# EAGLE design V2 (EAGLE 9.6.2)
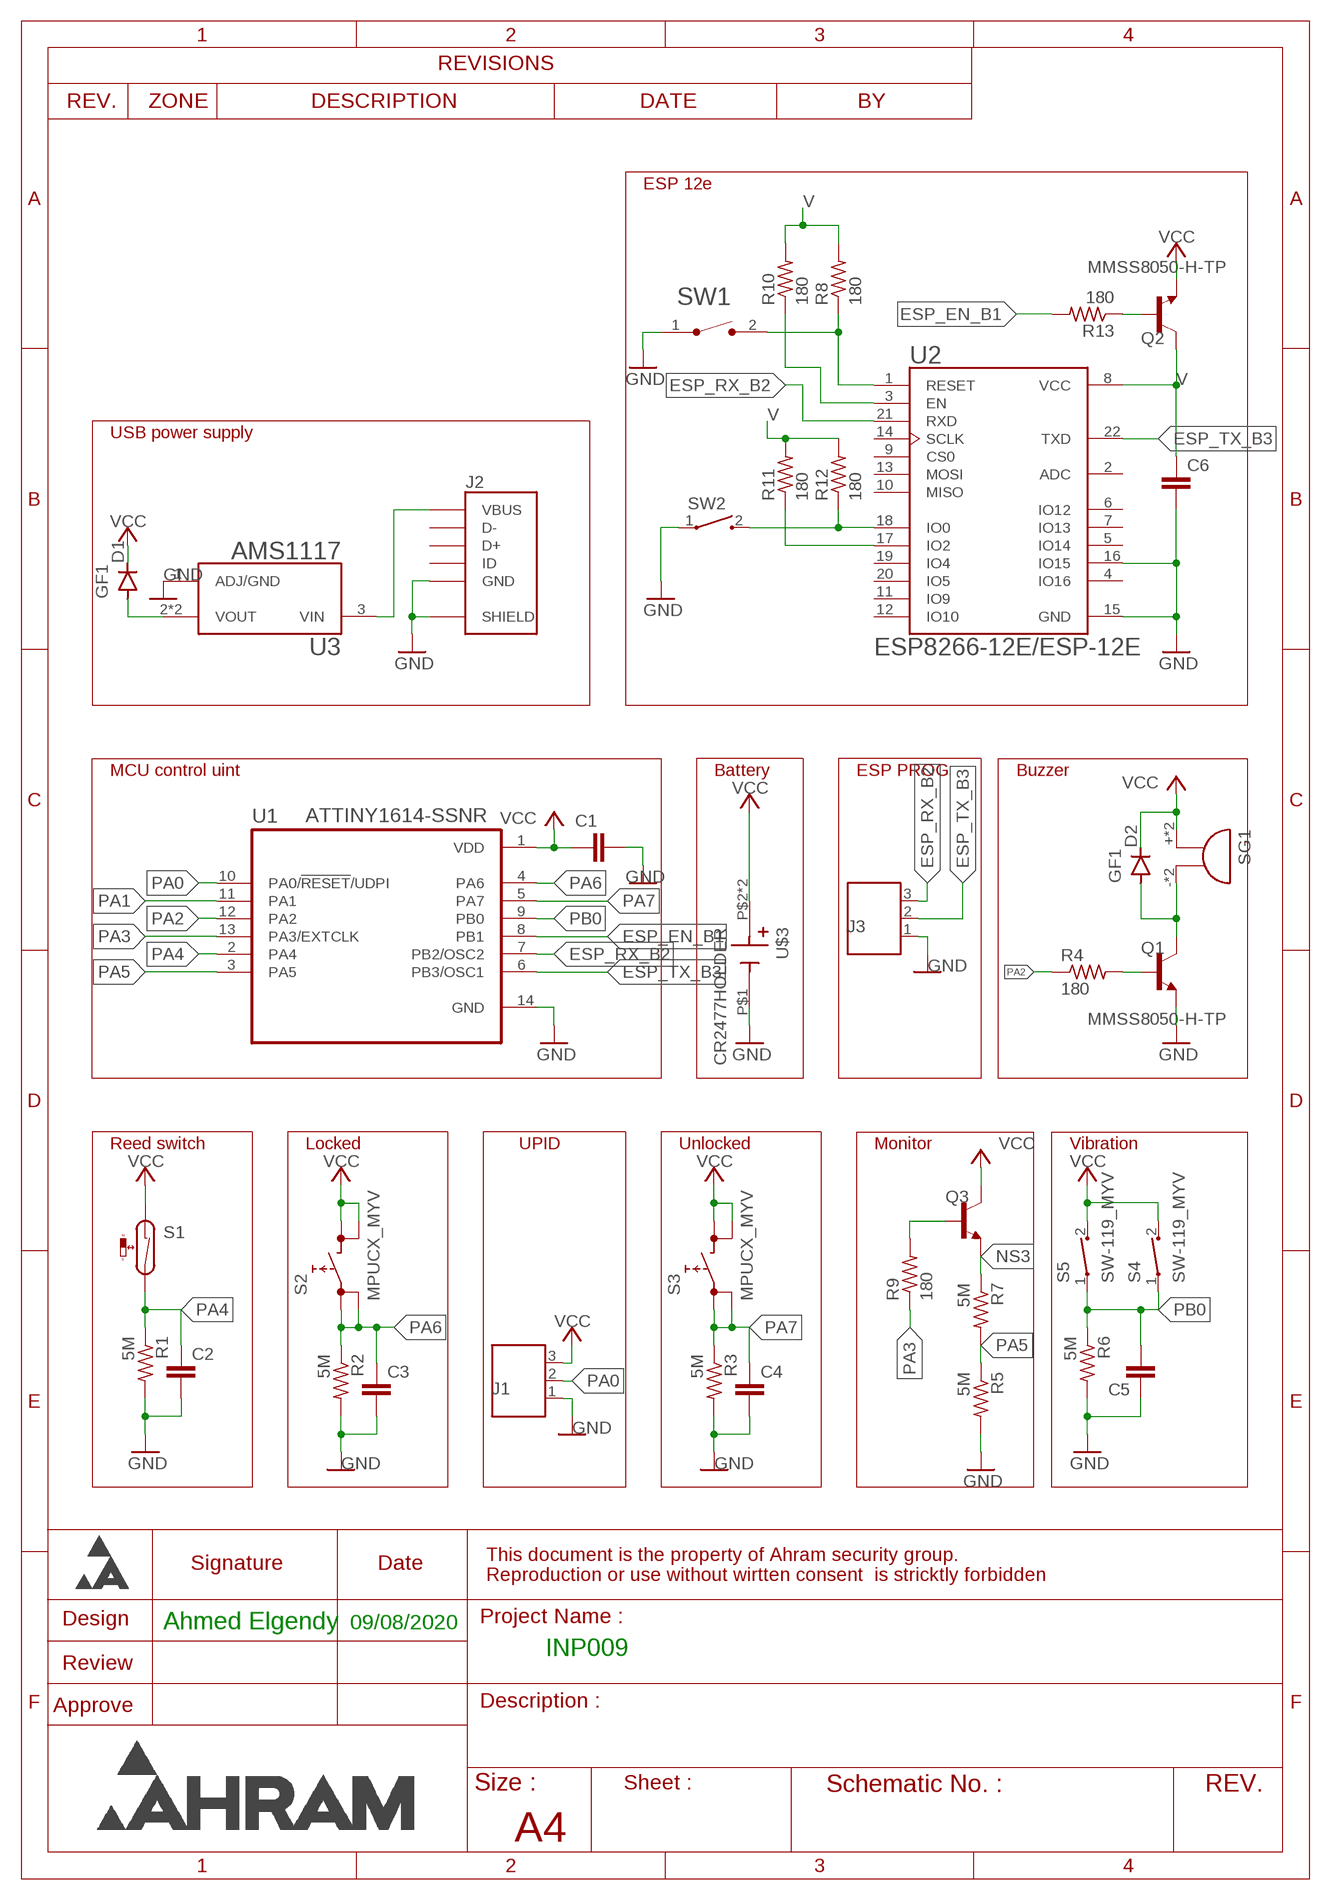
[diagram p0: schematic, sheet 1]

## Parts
C1  C-EUC0805K  [C0805K]
C2  C-EUC0805K  [C0805K]
C3  C-EUC0805K  [C0805K]
C4  C-EUC0805K  [C0805K]
C5  C-EUC0805K  [C0805K]
C6  C-EUC0805K  [C0805K]
D1  GF1  [SMA-DO214AC]
D2  GF1  [SMA-DO214AC]
J1  691508110303  [691508110303]
J2  USB3065-XX-00-A_REVE  [GCT_USB3065-XX-00-A_REVE]
J3  691508110303  [691508110303]
Q1  MMSS8050-H-TP  [TRANS_MMSS8050-H-TP]
Q2  MMSS8050-H-TP  [TRANS_MMSS8050-H-TP]
Q3  MMSS8050-H-TP  [TRANS_MMSS8050-H-TP]
R1  5M  R-US_M0805  [M0805]
R2  5M  R-US_M0805  [M0805]
R3  5M  R-US_M0805  [M0805]
R4  180  R-US_M0805  [M0805]
R5  5M  R-US_M0805  [M0805]
R6  5M  R-US_M0805  [M0805]
R7  5M  R-US_M0805  [M0805]
R8  180  R-US_M0805  [M0805]
R9  180  R-US_M0805  [M0805]
R10  180  R-US_M0805  [M0805]
R11  180  R-US_M0805  [M0805]
R12  180  R-US_M0805  [M0805]
R13  180  R-US_M0805  [M0805]
S1  RI80SMDM-MYV  [RI80SMDM-0510-J1]
S2  MPUCX_MYV  [MPUCX_MYV]
S3  MPUCX_MYV  [MPUCX_MYV]
S4  SW-119_MYV  [SW-119]
S5  SW-119_MYV  [SW-119]
SG1  CMI-9653S-SMT  [SMD_BUZZER]
SW1  FSMSM  [TE_FSMSM]
SW2  1437566-3  [SW_1437566-3]
U1  ATTINY1614-SSNR  [SOIC127P600X175-14N]
U2  ESP8266-12E/ESP-12E  [XCVR_ESP8266-12E/ESP-12E]
U3  AMS1117  [SOT229P700X180-4N]
U$3  CR2477HOLDER  [CR2477]

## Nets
ESP_EN_B1: R13.2 U1.8(PB1)
ESP_RX_B2: J3.3 U1.7(PB2/OSC2) U2.21(RXD)
ESP_TX_B3: J3.2 U1.6(PB3/OSC1) U2.22(TXD)
GND: C1.2 C2.2 C3.2 C4.2 C5.1 C6.2 J1.1 J2.5(GND) J2.6(SHIELD) J2.7(SHIELD) J2.8(SHIELD) J2.9(SHIELD) J3.1 Q1.2(E) R1.2 R2.2 R3.2 R5.2 R6.2 SW1.1 SW2.1 U1.14(GND) U2.15(GND) U2.16(IO15) U3.1(ADJ/GND) U$3.P$1(-)
N$2: D2.A Q1.3(C) SG1.- SG1.--(-)
N$3: J2.1(VBUS) U3.3(VIN)
N$4: Q1.1(B) R4.2
N$5: D1.A U3.2(VOUT) U3.4(VOUT)
N$6: Q3.1(B) R9.2
N$7: Q2.1(B) R13.1
N$9: R12.1 SW2.2 U2.18(IO0)
N$10: R11.1 U2.17(IO2)
N$11: R10.1 U2.3(EN)
N$12: R8.1 SW1.2 U2.1(RESET)
NS3: Q3.2(E) R7.1
PA0: J1.2 U1.10(PA0/!RESET!/UDPI)
PA1: U1.11(PA1)
PA2: R4.1 U1.12(PA2)
PA3: R9.1 U1.13(PA3/EXTCLK)
PA4: C2.1 R1.1 S1.P$2 U1.2(PA4)
PA5: R5.1 R7.2 U1.3(PA5)
PA6: C3.1 R2.1 S2.1 S2.2 U1.4(PA6)
PA7: C4.1 R3.1 S3.1 S3.2 U1.5(PA7)
PB0: C5.2 R6.1 S4.1 S5.1 U1.9(PB0)
V: C6.1 Q2.3(C) R8.2 R10.2 R11.2 R12.2 U2.8(VCC)
VCC: C1.1 D1.K(C) D2.K(C) J1.3 Q2.2(E) Q3.3(C) S1.P$1 S2.3 S2.4 S3.3 S3.4 S4.2 S5.2 SG1.+ SG1.++(+) U1.1(VDD) U$3.P$2(+) U$3.P$3(+)
Unconnected: J2.2(D-) J2.3(D+) J2.4(ID) U2.2(ADC) U2.4(IO16) U2.5(IO14) U2.6(IO12) U2.7(IO13) U2.9(CS0) U2.10(MISO) U2.11(IO9) U2.12(IO10) U2.13(MOSI) U2.14(SCLK) U2.19(IO4) U2.20(IO5)

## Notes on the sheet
- ESP 12e
- USB power supply
- MCU control uint | Battery | ESP PROG | Buzzer
- Reed switch | Locked | UPID | Unlocked | Monitor | Vibration
- Ahmed Elgendy | 09/08/2020
- INP009

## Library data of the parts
C1-C6 = rcl:C-EU: CAPACITOR, European symbol; SPICEPREFIX: C
D1 D2 = diode:GF1: DIODE
J1 J3 = Wurth_Elektronik_Electromechanic_Terminal_Blocks_Connectors_rev16b:691508110303: WR-TBL Terminal block - serie 5081 - 3 Pins;=>Code : Con_TBL_Screw_PClamp_3.50_6915081103xx_691508110303 Details see: http://katalog.we-online.de/em/datasheet/6915081103xx.pdf Created 11/3/2014, Karrer Zheng 2014 (C) Wurth Elektronik
J2 = USB3065-XX-00-A_REVE:USB3065-XX-00-A_REVE: Micro USB Receptacle, Type B, 5 Pin, SMT, Horizontal, Bottom Mount (Standart), Optional Plastic Locating Peg; AVAILABILITY: Unavailable; DESCRIPTION: USB3065 Series 5 Pin, SMT, Horizontal, Bottom Mount, Micro USB Receptacle; MF: Global Connector Technology; MP: USB3065-30-00-A; PACKAGE: None; PRICE: None
Q1-Q3 = MMSS8050-H-TP:MMSS8050-H-TP: MMSS8050-H Series 25 V 1.5 A NPN Silicon Plastic-Encapsulate Transistor-SOT-23; AVAILABILITY: Unavailable; DESCRIPTION: Bipolar _BJT_ Transistor NPN 25V 1.5A 100MHz 625mW Surface Mount SOT-23; MF: Micro Commercial; MP: MMSS8050-H-TP; PACKAGE: SOT-23 Micro Commercial; PRICE: None
R1-R13 = rcl:R-US_: RESISTOR, American symbol; SPICEPREFIX: R
S1 = reed_MYV:RI80SMDM-MYV
S2 S3 = shouhan_BP:MPUCX_MYV
S4 S5 = sw-119_MYV:SW-119_MYV
SG1 = CUI audio device:CMI-9653S-SMT
SW1 = FSMSM:FSMSM: Switch Tactile OFF (ON) SPST Rectangular Button Gull Wing 0.05A 12VDC SMD Loose Piece Check prices; AVAILABILITY: Warning; COMMENT: 1437566-3; CONFIGURATION_POLE-THROW: Single Pole - Single Throw; CONTACT_CURRENT_RATING: 50 mA; DESCRIPTION: Tactile Switch SPST-NO Top Actuated Surface Mount; MF: TE Connectivity; MP: FSMSM; PACKAGE: None; PRICE: None
SW2 = 1437566-3:1437566-3: Switch Tactile OFF (ON) SPST Rectangular Button Gull Wing 0.05A 12VDC SMD Loose Piece Check prices; AVAILABILITY: Warning; COMMENT: 1437566-3; CONFIGURATION_POLE-THROW: Single Pole - Single Throw; CONTACT_CURRENT_RATING: 50 mA; DESCRIPTION: Tactile Switch SPST-NO Top Actuated Surface Mount; MF: TE Connectivity; MP: 1437566-3; PACKAGE: None; PRICE: None
U1 = ATTINY1614-SSNR:ATTINY1614-SSNR: 20MHz, SOIC, 85C, Green, 14 SOIC .150in T/R; ARROW_ELECTRONICS-PURCHASE-URL: https://snapeda.com/shop?store=Arrow+Electronics&id=4817174; AVAILABILITY: Unavailable; DESCRIPTION: IC MCU 8BIT 16KB FLASH 14SOIC; DIGIKEY-PURCHASE-URL: https://snapeda.com/shop?store=DigiKey&id=4817174; MF: Microchip Technology; MOUSER-PURCHASE-URL: https://snapeda.com/shop?store=Mouser&id=4817174; MP: ATTINY1614-SSNR; PACKAGE: None; PRICE: None
U2 = ESP8266-12E_ESP-12E:ESP8266-12E/ESP-12E: ESP-12E WiFi Module; AVAILABILITY: Unavailable; DESCRIPTION: This WiFi module has a 32-bit MCU micro and clock speeds supporting 80 MHz or 160 MHz. Supports the RTOS and integrated Wi-Fi MAC/BB/RF/PA/LNA, and has an on-board antenna.; MF: AI-Thinker; MP: ESP8266-12E/ESP-12E; PACKAGE: None; PRICE: None
U3 = AMS1117:AMS1117: Sot223/Pkg 1-Amp 5-Volt Low Drop Out Voltage Regulatator; AVAILABILITY: Unavailable; DESCRIPTION: UNO PLUS Arduino R3 Shield, Xbee Arduino IDE Wheeled Robotics Kit; MF: Seeed Technology; MP: AMS1117; PACKAGE: SOT-223 Seeed Technology; PRICE: None
U$3 = cr2477_MYV:CR2477HOLDER

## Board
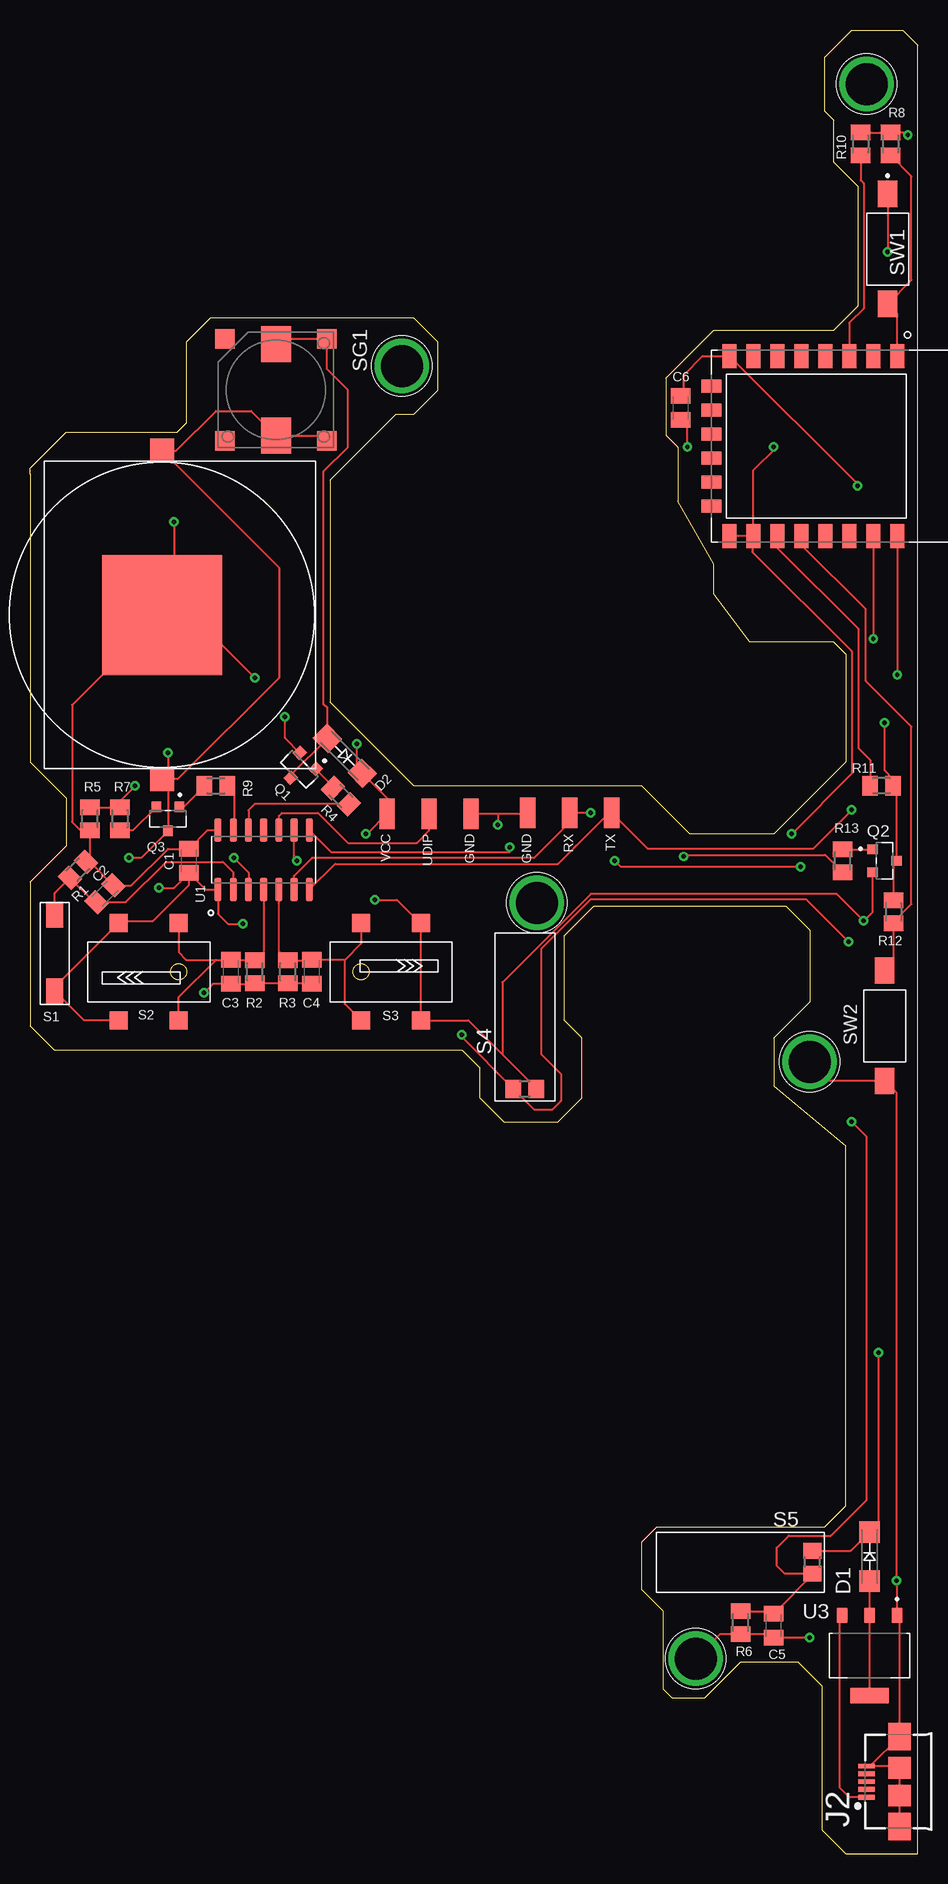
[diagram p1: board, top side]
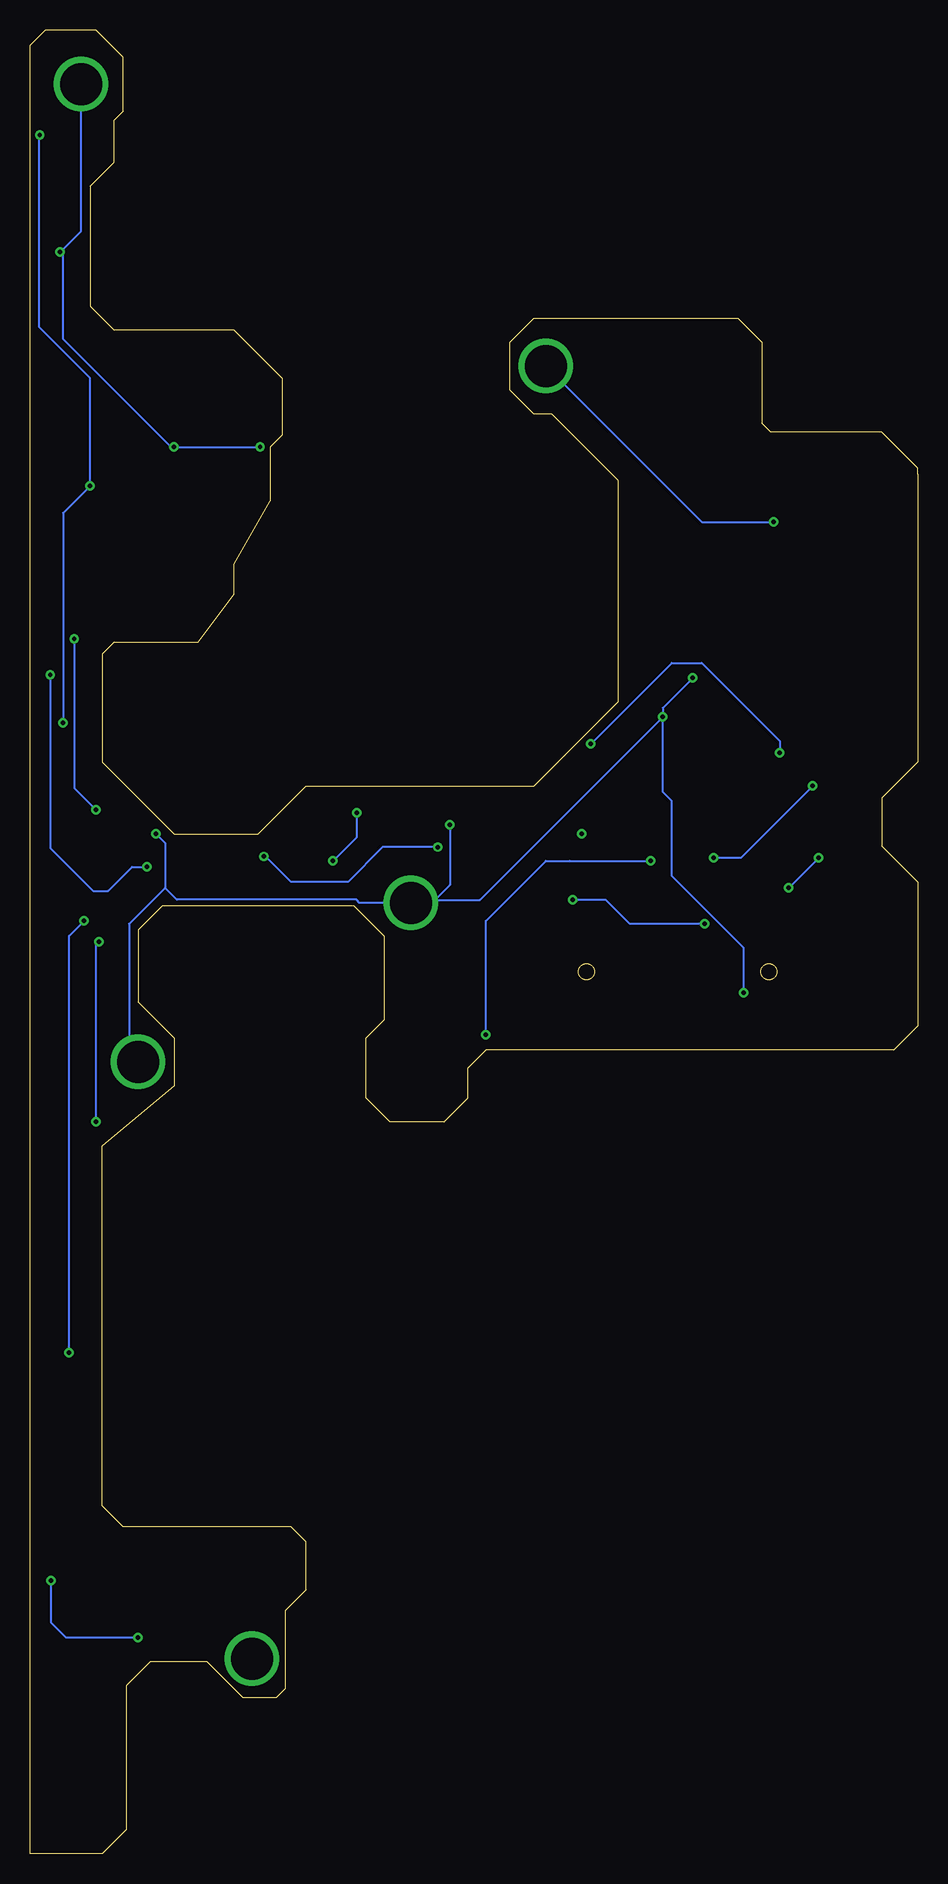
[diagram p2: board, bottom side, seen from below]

Size 74 x 152 mm. Coordinates in mm from the lower left corner, seen from the top.
Outline: 78 segments
Outline: circle at 12.4,73.5 radius 0.65
Outline: circle at 27.6,73.5 radius 0.65
Copper layers (1*16): Top 0.035mm / dielectric 1.5mm / Bottom 0.035mm
Design rules "default *": minimum track width 6mil, minimum drill 0.35mm, track to track 7mil, track to pad 7mil, pad to pad 7mil, via to via 7mil, smd to smd 7mil, copper to edge 15mil, drill to drill 6mil, minimum pad ring 10mil, minimum via ring 8mil, stop-mask expansion 4mil, vias tented up to drill 0mil, thermal gap 10mil

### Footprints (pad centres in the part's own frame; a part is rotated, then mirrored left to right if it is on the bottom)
C0805K = smd 1.3 x 1.6: 1 -1,0; 2 1,0
SMA-DO214AC = smd 1.8 x 1.7: A -2.05,0; K 2.05,0
691508110303 = smd 1.27 x 2.54: 1 -3.5,0; 2 0,0; 3 3.5,0
GCT_USB3065-XX-00-A_REVE = smd 0.4 x 1.4: 1 -1.3,0.5; 2 -0.65,0.5; 3 0,0.5; 4 0.65,0.5; 5 1.3,0.5 | smd 1.8 x 1.9: 6 1.15,-2.25; 7 -1.15,-2.25 | smd 2.3 x 1.9: 8 3.75,-2.25; 9 -3.75,-2.25
TRANS_MMSS8050-H-TP = smd 0.9 x 0.8: 1 -1,0.95; 2 -1,-0.95; 3 1,0
M0805 = smd 1.3 x 1.6: 1 -0.95,0; 2 0.95,0
RI80SMDM-0510-J1 = smd 2.1 x 1.45: P$1 -3,0; P$2 3.35,0
MPUCX_MYV = smd 1.5 x 1.5: 1 0.1,1.55; 2 0.1,-6.55; 3 5.1,1.55; 4 5.1,-6.55
SW-119 = smd 1.3 x 1.5: 1 -0.95,0; 2 0.95,0
SMD_BUZZER = smd 3 x 2.5: + 3.8,0; - -3.8,0 | smd 1.6 x 1.6: ++ 4.25,4.25; -- -4.25,4.25; N 4.25,-4.25; NC -4.25,-4.25
TE_FSMSM = smd 2.19 x 1.6: 1 -4.59,0; 2 4.59,0
SW_1437566-3 = smd 2.18 x 1.6: 1 -4.6,0; 2 4.6,0
SOIC127P600X175-14N = smd 1.95 x 0.59: 1 -2.48,3.81; 2 -2.48,2.54; 3 -2.48,1.27; 4 -2.48,0; 5 -2.48,-1.27; 6 -2.48,-2.54; 7 -2.48,-3.81; 8 2.48,-3.81; 9 2.48,-2.54; 10 2.48,-1.27; 11 2.48,0; 12 2.48,1.27; 13 2.48,2.54; 14 2.48,3.81
XCVR_ESP8266-12E/ESP-12E = smd 2 x 1.2: 1 -7.5,7; 2 -7.5,5; 3 -7.5,3; 4 -7.5,1; 5 -7.5,-1; 6 -7.5,-3; 7 -7.5,-5; 8 -7.5,-7; 15 7.5,-7; 16 7.5,-5; 17 7.5,-3; 18 7.5,-1; 19 7.5,1; 20 7.5,3; 21 7.5,5; 22 7.5,7 | smd 1.1 x 1.7: 9 -5,-8.5; 10 -3,-8.5; 11 -1,-8.5; 12 1,-8.5; 13 3,-8.5; 14 5,-8.5
SOT229P700X180-4N = smd 1.31 x 0.93: 1 -3.345,2.29; 2 -3.345,0; 3 -3.345,-2.29 | smd 1.31 x 3.24: 4 3.345,0
CR2477 = smd 10 x 10: P$1 0,0 | smd 2 x 2: P$2 13.7,0; P$3 -13.7,0

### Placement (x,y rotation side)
C1  13.25,82.75 90 top
C2  6.25,80 45 top
C3  16.75,73.5 270 top
C4  23.5,73.5 270 top
C5  62,19 90 top
C6  54.25,120.5 270 top
D1  70,24.75 90 top
D2  26.25,91.5 315 top
J1  33.28,86.68 180 top
J2  70.25,6 90 top
J3  45,86.75 0 top
Q1  22.45,90.37 225 top
Q2  71.25,82.75 0 top
Q3  11.5,86.25 270 top
R1  4,82 45 top
R2  18.75,73.5 270 top
R3  21.5,73.5 270 top
R4  25.92,88.14 135 top
R5  5,86.25 270 top
R6  59.25,19.25 270 top
R7  7.5,86.25 90 top
R8  71.75,142.5 90 top
R9  15.5,89 180 top
R10  69.25,142.5 90 top
R11  71,89 0 top
R12  72,78.5 90 top
R13  67.75,82.75 270 top
S1  2.06,74.89 90 top
S2  12.5,71 180 top
S3  27.5,76 0 top
S4  41.25,63.75 0 top
S5  65.23,24.28 90 top
SG1  20.5,122 270 top
SW1  71.5,133.75 270 top
SW2  71.25,69 90 top
U1  19.48,82.83 90 top
U2  65.31,117.32 270 top
U3  70,16.5 270 top
U$3  11,103.25 90 top

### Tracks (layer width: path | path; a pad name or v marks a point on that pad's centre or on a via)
ESP_EN_B1  (via drill 0.35)
  Top 0.152: R13.2 66.3,83.25 54.63,83.25 v54.5,83.12 | U1.8 25.1,83.5 40,83.5 v40,83.88
  Bottom 0.152: v40,83.88 44.62,83.88 47.5,81 52.25,81 54.5,83.25 v54.5,83.12
ESP_RX_B2  (via drill 0.35)
  Top 0.152: U2.21 v70.31,101.25 | v68.5,87 65.25,83.75 51.5,83.75 48.62,86.62 | 48.62,86.62 J3.3 | U1.7 25.44,82.5 44,82.5 45.38,83.88 45.5,84 48.12,86.62 48.62,86.62
  Bottom 0.152: v70.31,101.25 70.31,88.81 v68.5,87
ESP_TX_B3  (via drill 0.35)
  Top 0.152: U2.22 v72.31,98.25 | v64.25,82.25 49.25,82.25 v48.75,82.75 | U1.6 22.02,81.5 23.52,83 42,83 45,86 J3.2 v46.75,86.75
  Bottom 0.152: v72.31,98.25 72.31,83.81 68.75,80.25 67.5,80.25 65.5,82.25 v64.25,82.25 | v48.75,82.75 46.75,84.75 v46.75,86.75
GND  (via drill 0.35, 3.5)
  Top 0.152: 5,85.25 5,83 R1.2 4.99,82.67 C2.2 8.46,80.71 11.5,83.75 C1.2 14.81,85.31 U1.14 | 5,85.25 R5.2 | C4.2 23.45,72.55 R3.2 R2.2 18.7,72.5 C3.2 15.25,72.5 v14.5,71.75 | SW1.1 v71.5,133.5 | v54.81,117.25 54.81,118.94 C6.2 | U2.16 U2.15 | U2.16 60.31,115.31 62.25,117.25 v62,117.25 | U2.16 60.23,109.74 60.23,108.49 68.51,100.21 68.51,90.01 v63.5,85 | v55.5,16.25 57.55,18.3 R6.2 61.7,18.3 C5.1 v65,18 | v65,66 66.6,64.4 SW2.1 72.25,63.4 v72.25,22.75 72.29,22.71 U3.1 72.5,19.64 J2.8 70.05,7.3 J2.5 72.35,7.3 J2.6 J2.7 J2.9 | J3.1 41.43,86.68 39,86.68 | U$3.P$1 13.5,103.25 v18.75,98 | U$3.P$1 3.5,95.75 3.5,86 4.25,85.25 5,85.25 | Q1.2 21.25,92.98 v21.25,94.75 | J1.1 39,86.68 | 39,86.68 v39,85.75 | v12,111 12,104.25 U$3.P$1
  Bottom 0.152: 71.25,133.25 71.25,126.25 62.25,117.25 v62,117.25 v54.81,117.25 | 71.25,133.25 71.25,133.75 69.75,135.25 v69.75,147.5 | v65,18 71,18 72.25,19.25 v72.25,22.75 | v63.5,85 62.75,84.25 62.75,80.5 | v65,66 65.75,66.75 65.75,77.5 62.75,80.5 | v18.75,98 21.25,95.5 v21.25,94.75 | v14.5,71.75 14.5,75.5 20.5,81.5 20.5,87.75 21.25,88.5 v21.25,94.75 | 62.75,80.5 61.76,79.51 46.79,79.51 46.53,79.25 v42.25,79.25 40.5,79.25 40.25,79.5 | 40.25,79.5 36.5,79.5 v21.25,94.75 | v39,85.75 39,80.75 40.25,79.5 | v31,124 18,111 v12,111 | v71.5,133.5 71.25,133.25
N$2
  Top 0.152: Q1.3 21.74,89.89 D2.A 24.8,95.48 24.49,95.79 24.49,115.24 26.5,117.25 26.5,122 24.75,123.75 SG1.-- 20.5,126.25 20.25,126.5 20.25,126.05 SG1.-
N$3
  Top 0.152: J2.1 68.3,4.7 67.5,5.5 67.5,19.64 U3.3
N$4
  Top 0.152: Q1.1 25.25,88.99 R4.2
N$5
  Top 0.152: U3.4 U3.2 D1.A
N$6
  Top 0.152: Q3.1 12.8,87.25 R9.2
N$7
  Top 0.152: R13.1 Q2.1
N$9
  Top 0.152: U2.18 64.31,109.07 69.67,103.72 69.67,97.75 73.49,93.93 73.49,79.13 72,77.64 R12.1 72,74.35 SW2.2
N$10
  Top 0.152: U2.17 62.31,108.82 69.09,102.05 69.09,92.11 70.07,91.13 R11.1
N$11
  Top 0.152: U2.3 68.31,127.59 69.51,128.79 69.51,139.21 69.25,139.47 R10.1
N$12
  Top 0.152: R8.1 73.49,139.81 73.49,131.15 SW1.2 72.25,128.41 72.25,124.88 U2.1
NS3
  Top 0.152: R7.1 8.6,85.3 Q3.2
PA0
  Top 0.152: U1.10 20.75,86.5 21,86.75 24,86.75 26.5,84.25 32.25,84.25 33.28,85.28 J1.2
PA2
  Top 0.152: R4.1 18.72,87.47 18.21,86.96 U1.12
PA3
  Top 0.152: R9.1 17,88.45 17,84.5 16.94,84.56 U1.13
PA4
  Top 0.152: S1.P$2 2.06,80.06 R1.1 5.36,79.29 C2.1 7.98,79.29 11.34,82.65 16.1,82.65 16.94,81.81 U1.2
PA5  (via drill 0.35)
  Top 0.152: R5.1 R7.2 7.5,87.75 v8.75,89 | v17,83 18.21,81.79 U1.3
  Bottom 0.152: v8.75,89 14.75,83 v17,83
PA6
  Top 0.152: 15.5,74.5 13.04,74.5 12.4,75.14 S2.2 | 15.5,74.5 C3.1 18.7,74.5 R2.1 19.5,75.2 19.5,80.33 U1.4 | S2.1 12.4,71.4 15.5,74.5
PA7
  Top 0.152: S3.1 27.6,75.85 26.25,74.5 | 26.25,74.5 C4.1 23.45,74.45 R3.1 20.75,75.2 U1.5 | S3.2 26.25,70.8 26.25,74.5
PB0  (via drill 0.35)
  Top 0.152: R6.1 61.8,20.2 C5.2 65.23,23.23 S5.1 62.92,23.33 62.25,24 62.25,25.5 63.25,26.5 66.75,26.5 69.75,29.5 69.75,59.75 v68.5,61 | v68.25,76 64.74,79.51 46.72,79.51 42.61,75.39 42.61,66.64 44.25,65 44.25,62.75 43.5,62 42.05,62 S4.1 40.28,63.78 36,68.05 v36,68.25 | v22.25,82.75 22.02,82.98 U1.9
  Bottom 0.152: v68.5,61 68.5,75.75 v68.25,76 | v36,68.25 36,77.75 31,82.75 29,82.75 v22.25,82.75
V  (via drill 0.35)
  Top 0.152: R10.2 71.5,143.45 R8.2 72.99,143.45 v73.19,143.25 | C6.1 54.5,121.75 54.5,123.25 56.07,124.82 U2.8 69,114.13 v69,114 | R12.2 72,82.5 Q2.3 72.25,88.7 R11.2 71.95,89.57 71.25,90.27 v71.25,94.25
  Bottom 0.152: v71.25,94.25 71.25,111.75 v69,114 69,123 73.25,127.25 73.25,143.25 v73.19,143.25
VCC  (via drill 0.35)
  Top 0.152: S2.3 4.5,69.45 S1.P$1 2.06,72.21 S2.4 7.6,77.75 10.25,77.75 13.25,80.75 C1.1 | 32.6,77.5 S3.4 36.55,69.45 39.38,66.62 | 32.6,77.5 S3.3 | 11.15,89.4 U$3.P$3 12.3,89.55 20.75,98 20.75,107.2 U$3.P$2 12.2,116.95 15.5,120.25 18.45,120.25 SG1.+ 24.3,118.2 SG1.++ | 11.15,89.4 11.5,89.05 Q3.3 9.25,83 v8.25,83 | S5.2 68.43,25.23 D1.K 70.75,27.55 v70.75,41.75 | Q2.2 70.25,78.5 v69.5,77.75 67.25,80 46.75,80 39.38,72.62 39.38,66.62 | C1.1 14.65,80.35 U1.1 15.67,78.33 16.5,77.5 v17.75,77.5 | v10.75,80.5 12,80.5 C1.1 | 39.38,66.62 42.2,63.8 S4.2 | v28.75,79.5 30.6,79.5 32.6,77.5 | v28,85 28.1,85 J1.3 29.78,87.97 D2.K 27.25,90.5 v27.25,92.5 | v11.5,91.75 11.5,89.75 11.15,89.4
  Bottom 0.152: v70.75,41.75 70.75,76.5 v69.5,77.75 | v8.25,83 v10.75,80.5 | v17.75,77.5 24,77.5 26,79.5 v28.75,79.5 | v27.25,92.5 20.5,99.25 18,99.25 11.5,92.75 v11.5,91.75

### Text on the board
tNames: VCC | UDIP | GND | GND | RX | TX

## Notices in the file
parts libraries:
Wurth_Elektronik_Electromechanic_Termina: Copyright: Würth Elektronik
